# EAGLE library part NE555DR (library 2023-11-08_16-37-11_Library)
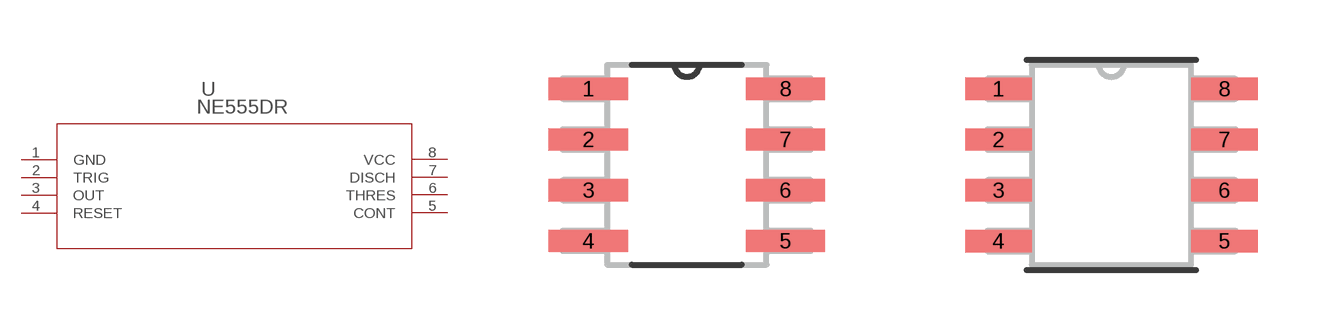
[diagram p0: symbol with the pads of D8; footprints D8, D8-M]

Designator prefix U

## NE555DRD8 (Copyright: Copyright (C) 2023 Ultra Librarian. All rights reserved.; Manufacturer_Part_Number: NE555DR; Mfr_Name: Texas Instruments)  [D8]
1  GND  pwr
2  TRIG  in
3  OUT  out
4  RESET  in
5  CONT  pas
6  THRES  in
7  DISCH  pas
8  VCC  pwr

## NE555DRD8-M (Copyright: Copyright (C) 2023 Ultra Librarian. All rights reserved.; Manufacturer_Part_Number: NE555DR; Mfr_Name: Texas Instruments)  [D8-M]
Pads as for D8

## NE555DRD8-L (Copyright: Copyright (C) 2023 Ultra Librarian. All rights reserved.; Manufacturer_Part_Number: NE555DR; Mfr_Name: Texas Instruments)  [D8-L]
Pads as for D8

## Footprint D8 (pad centres in mm)
smd 1.981 x 0.559: 1 -2.464,1.905; 2 -2.464,0.635; 3 -2.464,-0.635; 4 -2.464,-1.905; 5 2.464,-1.905; 6 2.464,-0.635; 7 2.464,0.635; 8 2.464,1.905

## Footprint D8-M (pad centres in mm)
smd 1.664 x 0.559: 1 -2.826,1.905; 2 -2.826,0.635; 3 -2.826,-0.635; 4 -2.826,-1.905; 5 2.826,-1.905; 6 2.826,-0.635; 7 2.826,0.635; 8 2.826,1.905

## Footprint D8-L (pad centres in mm)
smd 1.257 x 0.508: 1 -2.623,1.905; 2 -2.623,0.635; 3 -2.623,-0.635; 4 -2.623,-1.905; 5 2.623,-1.905; 6 2.623,-0.635; 7 2.623,0.635; 8 2.623,1.905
